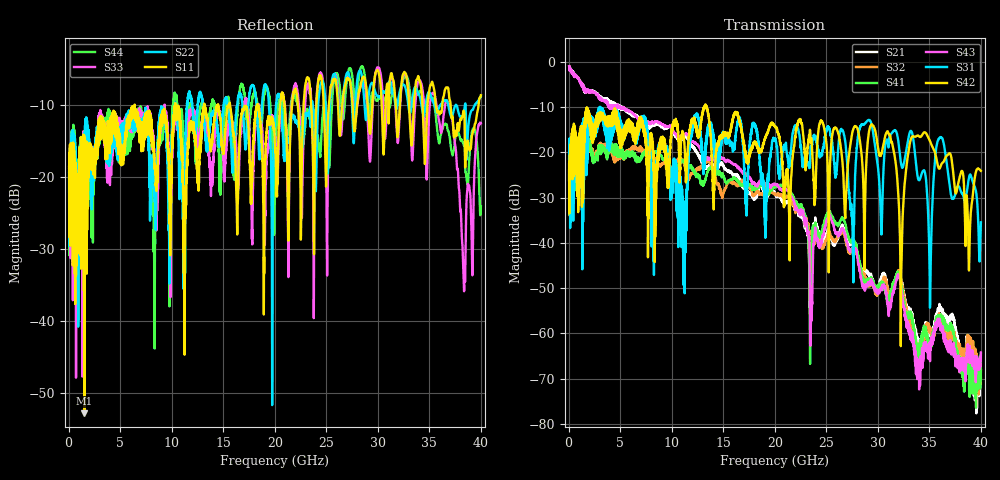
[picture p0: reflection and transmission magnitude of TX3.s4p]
!Agilent Technologies,N5245A,MY49151084,A.09.00.04
!Agilent N5245A: A.09.00.04
!Date: Thursday, January 20, 2011 09:01:01
!Correction: S11(Full 4 Port(1,2,3,4))
!S12(Full 4 Port(1,2,3,4))
!S13(Full 4 Port(1,2,3,4))
!S14(Full 4 Port(1,2,3,4))
!S21(Full 4 Port(1,2,3,4))
!S22(Full 4 Port(1,2,3,4))
!S23(Full 4 Port(1,2,3,4))
!S24(Full 4 Port(1,2,3,4))
!S31(Full 4 Port(1,2,3,4))
!S32(Full 4 Port(1,2,3,4))
!S33(Full 4 Port(1,2,3,4))
!S34(Full 4 Port(1,2,3,4))
!S41(Full 4 Port(1,2,3,4))
!S42(Full 4 Port(1,2,3,4))
!S43(Full 4 Port(1,2,3,4))
!S44(Full 4 Port(1,2,3,4))
!S4P File: Measurements: <S11,S12,S13,S14>,
!<S21,S22,S23,S24>,
!<S31,S32,S33,S34>,
!<S41,S42,S43,S44>:
# Hz S  dB  R 50
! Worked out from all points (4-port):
!   3996 points, 50 MHz to 40 GHz, reference 50 ohm
!   strongest paths, dB at 50 MHz, 10.04 GHz, 20.03 GHz, 30.02 GHz, 40 GHz:
!     S42: -22.6, -14.9, -14.3, -19.0, -24.1
!     S31: -21.4, -25.1, -16.9, -23.4, -35.5
!     S43: -1.0, -14.8, -27.0, -50.9, -64.2
!     S41: -26.0, -24.4, -27.5, -49.8, -64.4
!     S32: -26.1, -23.2, -29.3, -51.3, -69.8
!     S21: -0.9, -14.9, -29.0, -49.9, -68.2
!   lowest |S11| = -52.8 dB at 1.53 GHz (marker M1), VSWR 1.00, Z = 50 - j0.229 ohm
!   |S11| at or under -10 dB: start of sweep to 6.404 GHz; 6.411 GHz to 10.31 GHz (3.898 GHz wide, 46.6 % of centre); 10.35 GHz to 13.13 GHz (2.78 GHz wide, 23.7 % of centre)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
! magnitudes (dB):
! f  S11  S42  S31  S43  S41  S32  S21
! 50 MHz  -18.5  -22.6  -21.4  -1.0  -26.0  -26.1  -0.9
! 1.53 GHz  -52.8  -17.8  -24.1  -5.7  -16.8  -17.2  -5.7
! 27.51 GHz  -9.2  -15.8  -35.2  -41.7  -39.7  -41.3  -40.2
! 29.13 GHz  -12.2  -15.5  -12.8  -49.2  -48.4  -49.7  -47.1
! 32.25 GHz  -7.6  -51.6  -22.4  -49.7  -48.8  -48.1  -47.8
! 33.36 GHz  -14.2  -16.5  -16.0  -59.8  -57.2  -57.9  -55.9
! 40 GHz  -8.6  -24.1  -35.5  -64.2  -64.4  -69.8  -68.2
